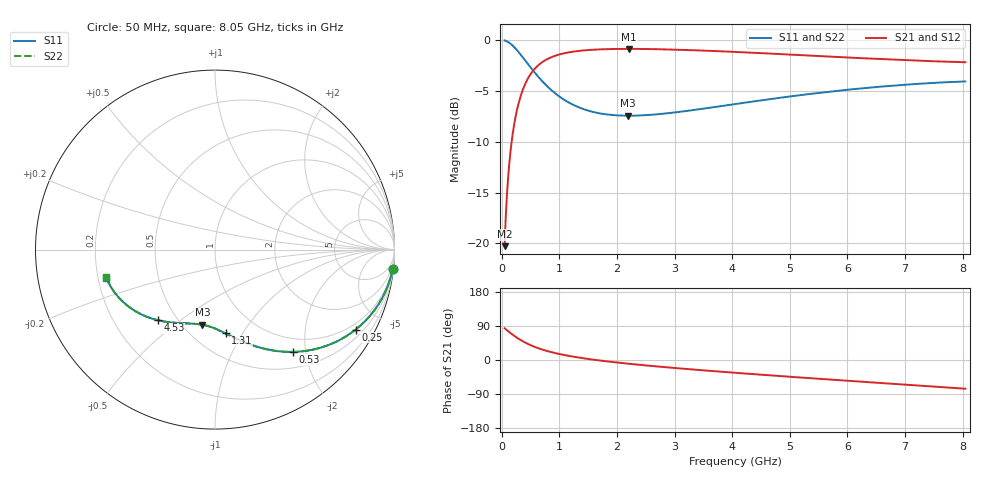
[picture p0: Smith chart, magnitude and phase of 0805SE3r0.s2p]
! AVX Thin Film Operation		Date: August 2001
! Description: Accu-P® Series, Thin Film, SMD, RF Capacitor
! Part Number: 08051J3R0ABT
! 50 MHz  -  8.05 GHz
! Serial Measurements
# mhz S db R 50
!	S11		S21		S12		S22
!	dB	Phase	dB	Phase	dB	Phase	dB	Phase
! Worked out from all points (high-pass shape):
!   401 points, 50 MHz to 8.05 GHz, reference 50 ohm
!   highest |S21| = -0.87 dB at 2.21 GHz (marker M1); lowest = -20.3 dB at 50 MHz (marker M2)
!   |S21| within 3 dB of the highest: 446.8 MHz to end of sweep
!   lowest |S11| = -7.4 dB at 2.19 GHz (marker M3), VSWR 2.47, Z = 31 - j31.7 ohm
!   |S11| at or under -10 dB: nowhere
!   |S22| runs from -7.4 to 0.0 dB; largest |S21 - S12| = 0
!   S11 on the Smith chart (normalised r, x): 50 MHz: 1, -18; 250 MHz: 0.76, -3.63; 530 MHz: 0.75, -1.77; 1.31 GHz: 0.71, -0.85; 4.53 GHz: 0.39, -0.42; 8.05 GHz: 0.23, -0.12
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50  -0.04 -6.4  -20.28 83.6  -20.28 83.6  -0.04 -6.4
70  -0.08 -8.9  -17.40 81.1  -17.40 81.1  -0.08 -8.9
110  -0.19 -13.8  -13.60 76.2  -13.60 76.2  -0.19 -13.8
150  -0.35 -18.6  -11.09 71.4  -11.09 71.4  -0.35 -18.6
190  -0.55 -23.2  -9.25 66.8  -9.25 66.8  -0.55 -23.2
250  -0.90 -29.7  -7.27 60.3  -7.27 60.3  -0.90 -29.7
370  -1.73 -40.9  -4.83 49.1  -4.83 49.1  -1.73 -40.9
530  -2.90 -52.7  -3.13 37.2  -3.13 37.2  -2.90 -52.8
690  -3.97 -61.7  -2.23 28.2  -2.23 28.2  -3.97 -61.8
850  -4.87 -68.8  -1.72 21.2  -1.72 21.2  -4.87 -68.8
1050  -5.75 -75.7  -1.35 14.2  -1.35 14.2  -5.75 -75.8
1310  -6.55 -82.8  -1.09 7.1  -1.09 7.1  -6.55 -82.9
1390  -6.74 -84.7  -1.04 5.2  -1.04 5.2  -6.74 -84.8
1750  -7.26 -92.1  -0.91 -2.2  -0.91 -2.2  -7.26 -92.2
2190  -7.45 -99.6  -0.87 -9.7  -0.87 -9.7  -7.45 -99.6
2210  -7.45 -99.9  -0.87 -10.0  -0.87 -10.0  -7.45 -99.9
2730  -7.29 -107.4  -0.90 -17.5  -0.90 -17.5  -7.29 -107.4
4050  -6.30 -123.6  -1.17 -33.7  -1.17 -33.7  -6.30 -123.7
4530  -5.91 -129.0  -1.29 -39.1  -1.29 -39.1  -5.91 -129.0
5390  -5.28 -138.2  -1.54 -48.4  -1.54 -48.4  -5.28 -138.3
6730  -4.51 -152.1  -1.91 -62.2  -1.91 -62.2  -4.51 -152.1
8050  -4.07 -165.6  -2.18 -75.8  -2.18 -75.8  -4.07 -165.7
